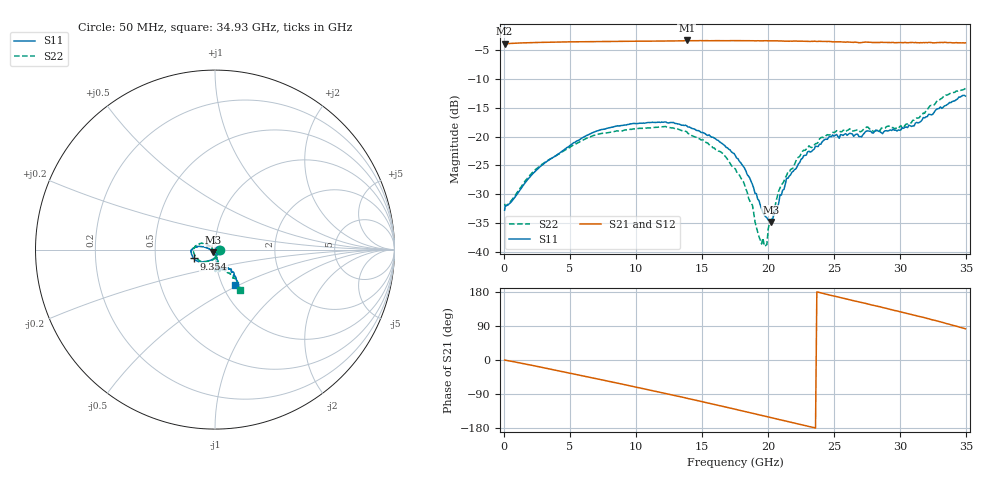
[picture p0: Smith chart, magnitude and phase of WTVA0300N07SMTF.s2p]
! 50 ohm 2-Port S-parameters measured by Modelithics Inc support@modelithics.com  Tampa, FL USA 813-866-6335 (February 2024)
! Smiths Interconnect,  3dB P/N: WTVA0300N07SMTF, Temperature: 0 C
! Board: 10 mil Rogers 4350B, Mounting Pad Dimensions: Length: 15 mils, Width: 25 mils, Gap: 40 mils.
# Hz S RI R 50
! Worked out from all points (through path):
!   352 points, 50 MHz to 34.93 GHz, reference 50 ohm
!   highest |S21| = -3.26 dB at 13.83 GHz (marker M1); lowest = -3.8 dB at 50 MHz (marker M2)
!   group delay of S21, straight-line fit = 22 ps
!   lowest |S11| = -34.8 dB at 20.2 GHz (marker M3), VSWR 1.04, Z = 48.9 - j1.39 ohm
!   |S11| at or under -10 dB: start of sweep to end of sweep
!   |S22| runs from -39.0 to -11.6 dB; largest |S21 - S12| = 0.0044
!   S11 on the Smith chart (normalised r, x): 50 MHz: 1.05, -0.00; 9.354 GHz: 0.79, -0.08; 34.93 GHz: 1.15, -0.47
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5e7  0.0229 -0.00165  0.6436 -0.00266  0.6436 -0.00297  0.0261 -0.00151
2.6875e9  -0.0113 -0.053  0.6279 -0.2051  0.6275 -0.2051  -0.00818 -0.0549
5.8715e9  -0.0685 -0.0686  0.5043 -0.4403  0.5039 -0.4403  -0.0629 -0.0674
9.354e9  -0.1177 -0.0495  0.2665 -0.6201  0.2658 -0.62  -0.1079 -0.04
1.1742e10  -0.1328 -0.0168  0.062 -0.6758  0.0611 -0.6757  -0.1216 -0.00874
1.38315e10  -0.1243 0.00687  -0.1285 -0.6749  -0.1287 -0.6746  -0.1085 0.0217
1.7513e10  -0.0666 0.0166  -0.4415 -0.5244  -0.4418 -0.5239  -0.0444 0.0283
1.88065e10  -0.038 0.00638  -0.528 -0.4348  -0.5278 -0.4345  -0.0232 0.0103
1.9503e10  -0.0234 -0.00231  -0.5661 -0.3795  -0.566 -0.3793  -0.0111 -0.00363
1.96025e10  -0.0215 -0.00385  -0.5716 -0.3733  -0.5712 -0.3734  -0.0113 -0.00678
1.9901e10  -0.0173 -0.00957  -0.5877 -0.3467  -0.5872 -0.3469  -0.00472 -0.0105
2.00005e10  -0.0153 -0.0111  -0.5924 -0.3383  -0.5919 -0.3386  -0.00454 -0.0151
2.01995e10  -0.0112 -0.0142  -0.6018 -0.321  -0.6014 -0.321  -0.00443 -0.0175
2.07965e10  0.000651 -0.0264  -0.6252 -0.2669  -0.6252 -0.2661  0.00562 -0.0333
2.1493e10  0.00436 -0.0433  -0.6457 -0.2045  -0.6456 -0.2039  0.0105 -0.0482
2.25875e10  0.0139 -0.0633  -0.6686 -0.1017  -0.6683 -0.1011  0.0183 -0.0722
2.33835e10  0.0121 -0.0756  -0.6743 -0.0271  -0.6741 -0.0268  0.0156 -0.08
2.4876e10  0.0152 -0.1025  -0.6571 0.1222  -0.6567 0.1226  0.00919 -0.1085
2.91545e10  0.0319 -0.1086  -0.4587 0.4739  -0.4578 0.4743  0.0237 -0.1215
3.01495e10  0.0574 -0.1048  -0.3866 0.5299  -0.386 0.53  0.0417 -0.111
3.33335e10  0.1112 -0.1479  -0.0899 0.6554  -0.0897 0.655  0.1298 -0.1882
3.49255e10  0.1117 -0.1962  0.0877 0.6488  0.0906 0.648  0.1389 -0.2236
